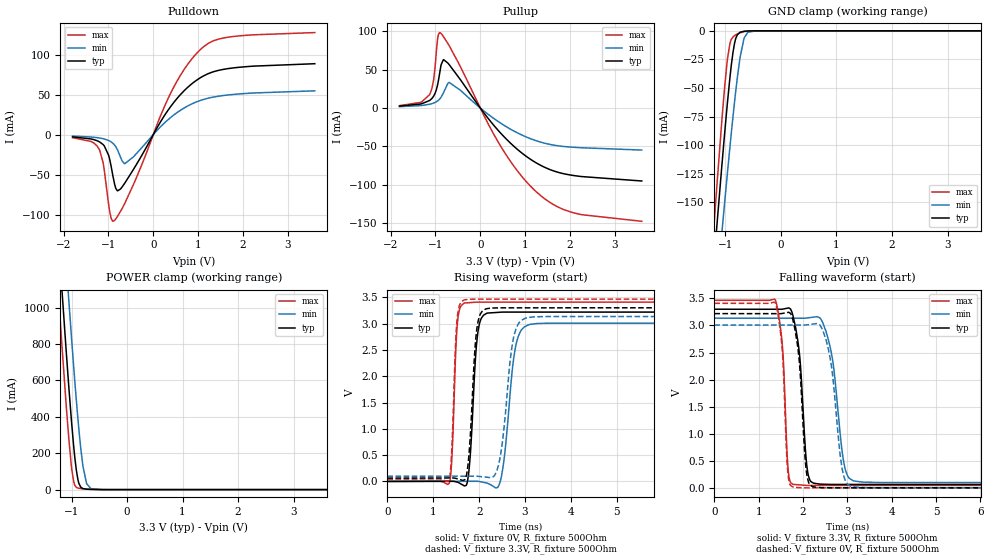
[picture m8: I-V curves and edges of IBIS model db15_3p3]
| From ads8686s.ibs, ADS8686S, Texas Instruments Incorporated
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|   db15_3p3 Model
[Model]   db15_3p3
Model_type   I/O
Polarity   Non-Inverting
Enable   Active-Low
Vinl = 0.99
Vinh = 2.31
Vmeas = 1.65
Vref = 1.65
Cref = 15pF
Rref = 50
|   typ   min   max
C_comp   1.51pF   1.51pF   1.55pF
[Voltage Range]   3.3   3.135   3.465
[Temperature Range]   27   125   -40
[Pullup Reference]   3.3   3.135   3.465
[Pulldown Reference]   0   -0   0
[Power Clamp Reference]   3.3   3.135   3.465
[GND Clamp Reference]   0   0   0
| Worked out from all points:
|   slope of the pulldown table from 0 to 0.495 V, typ, clamps not added: 11.6 ohm
|   slope of the pullup table from 0 to 0.495 V, typ, clamps not added: 14 ohm
|   GND clamp passes 1 mA (typ) near -0.72 V on its own axis
|   POWER clamp passes 1 mA (typ) near -0.62 V on its own axis
|   falling waveform, V_fixture 3.3V, R_fixture 500Ohm: 20-80 % time 160ps typ, 247ps min, 118ps max; typ from 3.3 V to 0.063 V
|   rising waveform, V_fixture 0V, R_fixture 500Ohm: 20-80 % time 123ps typ, 198ps min, 85.5ps max; typ from 0 V to 3.22 V
|   rising waveform, V_fixture 3.3V, R_fixture 500Ohm: 20-80 % time 125ps typ, 209ps min, 85.5ps max; typ from 0.063 V to 3.3 V
|   falling waveform, V_fixture 0V, R_fixture 500Ohm: 20-80 % time 153ps typ, 231ps min, 115ps max; typ from 3.22 V to 0 V
[Pulldown]
|   Voltage   I(typ)   I(min)   I(max)
-1.8V     -2.907mA   -1.879mA   -3.868mA
-1.39V    -5.481mA   -3.066mA   -8.598mA
-1.201V   -9.104mA   -4.303mA   -18.96mA
-1.114V   -12.84mA   -5.256mA   -36.8mA
-995.4mV  -26.08mA   -7.476mA   -87.72mA
-903.6mV  -50.95mA   -10.8mA    -108.5mA
-801mV    -70.28mA   -18.82mA   -102.5mA
-639mV    -60.99mA   -36.57mA   -86.38mA
387mV     35.03mA    21.36mA    51.79mA
1.046V    70.95mA    42.59mA    106.1mA
1.672V    82.52mA    49.55mA    121.8mA
3.6V      88.61mA    54.67mA    127.6mA
[GND Clamp]
|   Voltage   I(typ)   I(min)   I(max)
-1.8V     -575.1mA   -590.1mA   -589.5mA
-1.211V   -205.2mA   -256.8mA   -174.1mA
-1.152V   -169.4mA   -224.2mA   -134.4mA
-1.066V   -118.7mA   -177.6mA   -79.19mA
-1.017V   -91.27mA   -151.8mA   -50.81mA
-963mV    -62.4mA    -123.9mA   -24.53mA
-903.6mV  -34.11mA   -94.13mA   -8.664mA
-822.6mV  -8.191mA   -56.42mA   -3.809mA
-736.2mV  -1.24mA    -23.24mA   -1.747mA
-666mV    -402uA     -6.834mA   -720.4uA
-595.8mV  -133uA     -1.235mA   -229.3uA
3.6V      0A         0A         0A
[Pullup]
|   Voltage   I(typ)   I(min)   I(max)
-1.8V     2.405mA    1.644mA    3.009mA
-1.336V   5.083mA    3.038mA    7.181mA
-1.13V    9.67mA     4.794mA    17.2mA
-1.044V   14.98mA    6.27mA     35.17mA
-952.2mV  29.87mA    9.102mA    89.43mA
-903.6mV  45.93mA    11.68mA    98.43mA
-822.6mV  62.99mA    19.41mA    93.32mA
-693mV    56.58mA    33.35mA    81.43mA
387mV     -28.48mA   -17.22mA   -43.21mA
1.229V    -71.12mA   -42.47mA   -108.4mA
2.05V     -87.97mA   -51.25mA   -136.4mA
3.6V      -95.41mA   -55mA      -148mA
[POWER Clamp]
|   Voltage   I(typ)   I(min)   I(max)
-1.8V     4.061A     4.54A      3.768A
-1.233V   1.367A     1.858A     1.061A
-1.179V   1.123A     1.613A     817.9mA
-1.049V   564.5mA    1.04A      280.1mA
-995.4mV  355.2mA    812.6mA    109.9mA
-963mV    243.1mA    681mA      46.78mA
-914.4mV  108.2mA    493.5mA    12.79mA
-865.8mV  32.73mA    323.4mA    7.075mA
-795.6mV  5.598mA    130.2mA    4.664mA
-730.8mV  2.41mA     35.35mA    3.08mA
-649.8mV  1.154mA    4.788mA    1.533mA
3.6V      0A         0A         0A
[Ramp]
R_load = 500
|   typ   min   max
dV/dt_r   1.9313/1.22728e-10   1.80504/1.96814e-10   2.04523/8.54882e-11
dV/dt_f   1.94226/1.60003e-10   1.82241/2.4685e-10   2.05211/1.18479e-10
[Falling Waveform]
V_fixture = 3.3V
V_fixture_min = 3.135V
V_fixture_max = 3.465V
R_fixture = 500Ohm
C_fixture = 0F
|   Time   V(typ)   V(min)   V(max)
0s        3.3V       3.135V     3.465V
1.376ns   3.299V     3.134V     3.471V
1.544ns   3.302V     3.134V     2.529V
1.664ns   3.322V     3.134V     342.6mV
1.773ns   3.184V     3.134V     66.91mV
2.221ns   93.84mV    3.152V     45.09mV
2.593ns   64.26mV    2.67V      45.08mV
2.924ns   63.42mV    453.3mV    45.07mV
3.121ns   63.41mV    136.5mV    45.06mV
10ns      62.9mV     97.65mV    44.81mV
[Rising Waveform]
V_fixture = 0V
V_fixture_min = 0V
V_fixture_max = 0V
R_fixture = 500Ohm
C_fixture = 0F
|   Time   V(typ)   V(min)   V(max)
0s        -101.2nV   128.2nV    -47.71nV
1.348ns   2.918mV    1.619mV    -31.88mV
1.52ns    -13.07mV   1.825mV    2.945V
1.673ns   -82.56mV   2.009mV    3.389V
1.965ns   2.783V     2.359mV    3.409V
2.168ns   3.196V     -32.07mV   3.409V
2.468ns   3.216V     23.68mV    3.409V
2.789ns   3.219V     2.535V     3.409V
3.068ns   3.219V     2.974V     3.409V
10ns      3.219V     3.008V     3.409V
[Rising Waveform]
V_fixture = 3.3V
V_fixture_min = 3.135V
V_fixture_max = 3.465V
R_fixture = 500Ohm
C_fixture = 0F
|   Time   V(typ)   V(min)   V(max)
0s        62.9mV     97.65mV    44.81mV
1.34ns    65.59mV    99.18mV    23.6mV
1.512ns   52.87mV    99.38mV    3.001V
1.664ns   24.38mV    99.55mV    3.445V
1.951ns   2.903V     98.87mV    3.465V
2.138ns   3.276V     81.95mV    3.465V
2.418ns   3.298V     294.5mV    3.465V
2.743ns   3.3V       2.7V       3.465V
3.005ns   3.3V       3.101V     3.465V
10ns      3.3V       3.135V     3.465V
[Falling Waveform]
|Gnd
V_fixture = 0V
V_fixture_min = 0V
V_fixture_max = 0V
R_fixture = 500Ohm
C_fixture = 0F
|   Time   V(typ)   V(min)   V(max)
0s        3.219V     3.008V     3.409V
1.376ns   3.218V     3.008V     3.414V
1.536ns   3.222V     3.008V     2.499V
1.655ns   3.24V      3.008V     308.6mV
1.76ns    3.135V     3.008V     22.09mV
2.073ns   322.9mV    3.01V      478.4uV
2.205ns   26.71mV    3.024V     230.1uV
2.57ns    1.501mV    2.565V     219.4uV
3.068ns   346.3uV    32.74mV    204.7uV
10ns      49.63nV    355.1nV    -58.05nV
